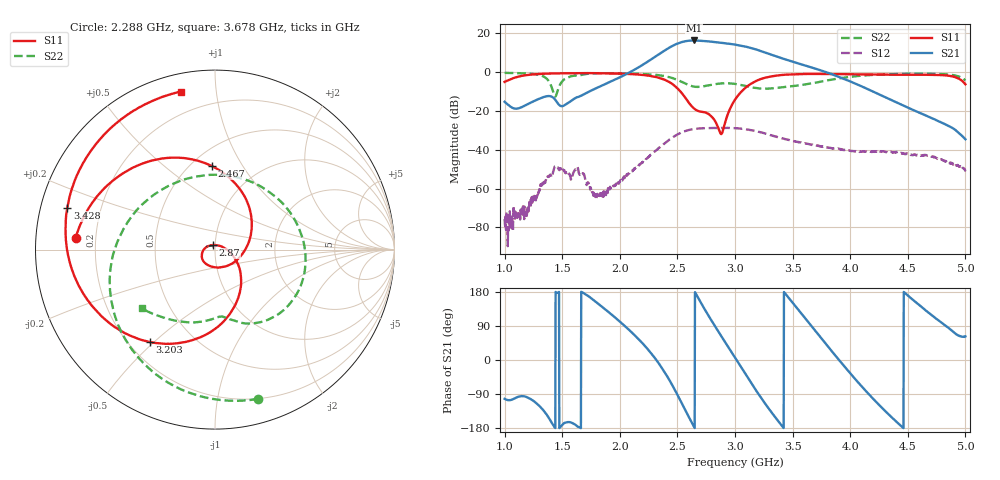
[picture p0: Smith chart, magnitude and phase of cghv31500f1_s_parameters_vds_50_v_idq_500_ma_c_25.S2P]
!Keysight Technologies,E5071C,MY46632031,B.14.03
!Date: Fri Jul 09 16:05:50 2021
!Data & Calibration Information:
!Freq	S11:SOLT2(ON)	S21:SOLT2(ON)	S12:SOLT2(ON)	S22:SOLT2(ON)
!PortZ  Port1:50+j0  Port2:50+j0
!Above PortZ is port z conversion or system Z0 setting when saving the data.
!When reading, reference impedance value at option line is always used.
# Hz S dB R 50
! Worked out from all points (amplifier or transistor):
!   1601 points, 1 GHz to 5 GHz, reference 50 ohm
!   highest |S21| = 16.3 dB at 2.645 GHz (marker M1)
!   |S21| within 3 dB of that: 2.451 GHz to 3.079 GHz (628.5 MHz wide, 22.7 % of centre)
!   unconditionally stable (mu >= 1): start of sweep to end of sweep
!   at 1.665 GHz: K = 25.47, MAG = 3.1 dB, |S12| = -52.4 dB
!   at 3 GHz: K = 1.96, MAG = 15.9 dB, |S12| = -28.9 dB
!   at 5 GHz: K = 4228.21, MAG = -31.4 dB, |S12| = -50.4 dB
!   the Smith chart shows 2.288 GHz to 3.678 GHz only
!   S11 on the Smith chart (normalised r, x): 2.288 GHz: 0.12, +0.04; 2.467 GHz: 0.63, +0.74; 2.87 GHz: 0.98, +0.05; 3.203 GHz: 0.28, -0.49; 3.428 GHz: 0.08, +0.14; 3.678 GHz: 0.09, +0.81
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1e9  -5.01 154.1  -15.27 -102.5  -75.70 138.7  -0.38 122.6
1.315e9  -0.90 75.4  -13.34 -125.3  -58.25 -128.1  -1.68 61.7
1.6675e9  -0.49 -15.3  -12.05 179.6  -52.44 -162.2  -1.43 55.0
2.04e9  -0.82 -109.1  -1.51 90.7  -54.66 7.8  -0.64 -16.9
2.2875e9  -2.17 175.0  7.16 11.8  -41.58 -71.2  -1.25 -73.9
2.335e9  -2.81 156.6  9.04 -7.5  -39.23 -91.1  -1.54 -88.3
2.4075e9  -4.40 124.0  11.83 -41.1  -35.87 -124.9  -2.25 -114.2
2.4675e9  -6.64 92.1  13.86 -73.0  -33.29 -156.8  -3.26 -141.0
2.55e9  -11.68 38.4  15.68 -121.2  -30.75 154.8  -5.37 173.6
2.645e9  -18.76 -49.7  16.33 -176.7  -29.27 99.5  -7.46 110.0
2.76e9  -21.21 -145.3  15.90 122.0  -28.81 38.3  -6.96 39.9
2.87e9  -31.06 113.7  15.19 68.2  -28.74 -15.5  -5.87 -7.6
3e9  -14.15 -43.2  14.20 6.2  -28.89 -77.3  -6.05 -48.6
3.1075e9  -7.26 -88.5  12.94 -45.2  -29.57 -128.3  -7.35 -71.1
3.2025e9  -4.02 -125.1  11.33 -89.3  -30.67 -171.8  -8.36 -81.4
3.3075e9  -2.25 -160.7  9.19 -134.2  -32.40 143.3  -8.40 -89.3
3.4275e9  -1.36 164.3  6.75 178.6  -34.33 96.4  -7.67 -102.5
3.6675e9  -0.91 104.4  2.36 88.3  -37.47 8.5  -5.73 -139.7
3.6775e9  -0.91 102.0  2.17 84.6  -37.47 5.0  -5.63 -141.5
3.995e9  -1.07 26.0  -4.64 -33.2  -40.43 -97.9  -2.45 143.6
4.335e9  -1.31 -65.5  -13.74 -143.8  -41.11 177.3  -1.06 63.0
5e9  -6.24 120.1  -34.59 62.3  -50.39 36.4  -4.26 -50.0
